(* Logix 5000 AddOnInstructionDefinition export SPEL_Above; software revision 30.01; part 3 of 9 *)

ADD_ON_INSTRUCTION SPEL_FineSet   (* revision 1.0, vendor SEIKO EPSON CORP. *)
// Sets the positioning end judgement range for all joints.
VAR_INPUT
   Start : BOOL; {required}
END_VAR
VAR_OUTPUT
   InCycle : BOOL; {access Read Only, visible}
   Done : BOOL; {access Read Only, visible}
   Error : BOOL; {access Read Only, visible}
END_VAR
VAR_INPUT
   Axis1 : DINT; {required}
   Axis2 : DINT; {required}
   Axis3 : DINT; {required}
   Axis4 : DINT; {required}
   Axis5 : DINT; {required}
   Axis6 : DINT; {required}
END_VAR
VAR_IN_OUT
   ExtInputs : AB:ETHERNET_MODULE_INT_128Bytes:I:0; {required}
   ExtOutputs : AB:ETHERNET_MODULE_INT_128Bytes:O:0; {required}
END_VAR
VAR_OUTPUT
   ErrCode1 : INT; {access Read Only, visible}
   ErrCode2 : INT; {access Read Only, visible}
END_VAR
VAR
   ExecFineSet : SPEL_ExecCmd := (MaxTime := 3000); {access None}
   OneShotStart : BOOL; {access None}
   StartCoil : BOOL; {access None}
   ExecTimeout : DINT; {access None}
END_VAR

ROUTINE Logic   (* ladder *)
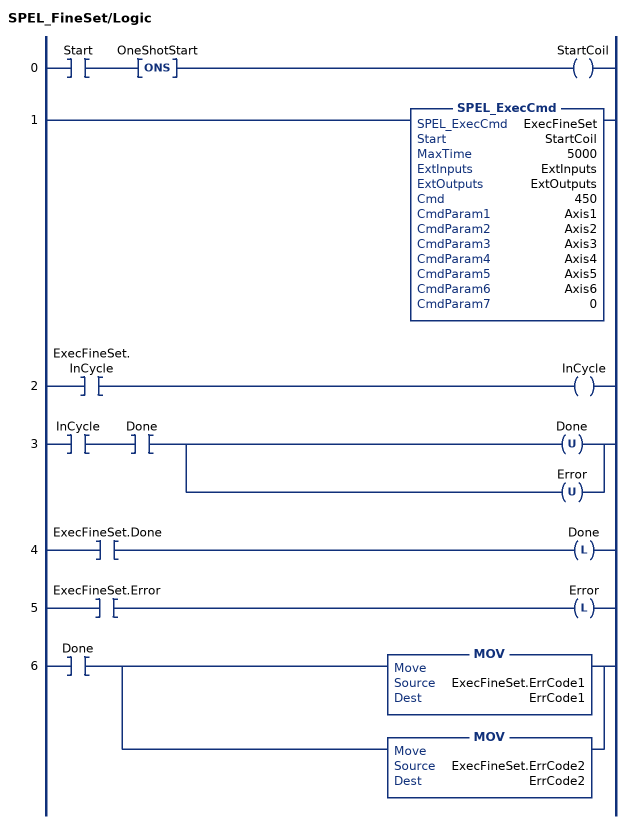
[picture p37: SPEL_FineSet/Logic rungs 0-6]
   0: XIC(Start)ONS(OneShotStart)OTE(StartCoil);
   1: SPEL_ExecCmd(ExecFineSet,StartCoil,5000,ExtInputs,ExtOutputs,450,Axis1,Axis2,Axis3,Axis4,Axis5,Axis6,0);
   2: XIC(ExecFineSet.InCycle)OTE(InCycle);
   3: XIC(InCycle)XIC(Done)[OTU(Done) ,OTU(Error) ];
   4: XIC(ExecFineSet.Done)OTL(Done);
   5: XIC(ExecFineSet.Error)OTL(Error);
   6: XIC(Done)[MOV(ExecFineSet.ErrCode1,ErrCode1) ,MOV(ExecFineSet.ErrCode2,ErrCode2) ];
END_ROUTINE
END_ADD_ON_INSTRUCTION

ADD_ON_INSTRUCTION SPEL_Flip   (* revision 1.0, vendor SEIKO EPSON CORP. *)
// Sets the wrist orientation of the specified point to Flip.
VAR_INPUT
   Start : BOOL; {required}
END_VAR
VAR_OUTPUT
   InCycle : BOOL; {access Read Only, visible}
   Done : BOOL; {access Read Only, visible}
   Error : BOOL; {access Read Only, visible}
END_VAR
VAR_INPUT
   Point : INT; {required}
END_VAR
VAR_IN_OUT
   ExtInputs : AB:ETHERNET_MODULE_INT_128Bytes:I:0; {required}
   ExtOutputs : AB:ETHERNET_MODULE_INT_128Bytes:O:0; {required}
END_VAR
VAR_OUTPUT
   ErrCode1 : INT; {access Read Only, visible}
   ErrCode2 : INT; {access Read Only, visible}
END_VAR
VAR
   ExecFlip : SPEL_ExecCmd := (MaxTime := 3000); {access None}
   OneShotStart : BOOL; {access None}
   StartCoil : BOOL; {access None}
   ExecTimeout : DINT; {access None}
END_VAR

ROUTINE Logic   (* ladder *)
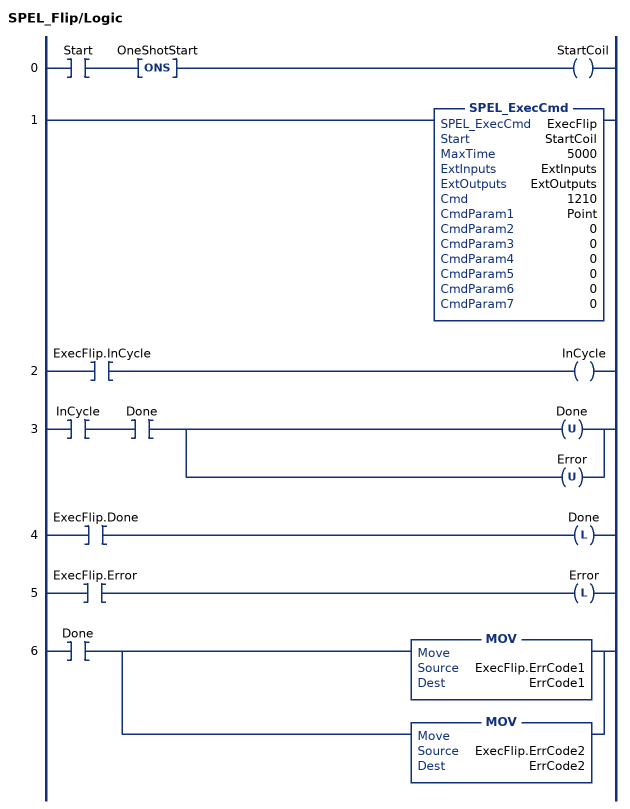
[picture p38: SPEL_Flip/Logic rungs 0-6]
   0: XIC(Start)ONS(OneShotStart)OTE(StartCoil);
   1: SPEL_ExecCmd(ExecFlip,StartCoil,5000,ExtInputs,ExtOutputs,1210,Point,0,0,0,0,0,0);
   2: XIC(ExecFlip.InCycle)OTE(InCycle);
   3: XIC(InCycle)XIC(Done)[OTU(Done) ,OTU(Error) ];
   4: XIC(ExecFlip.Done)OTL(Done);
   5: XIC(ExecFlip.Error)OTL(Error);
   6: XIC(Done)[MOV(ExecFlip.ErrCode1,ErrCode1) ,MOV(ExecFlip.ErrCode2,ErrCode2) ];
END_ROUTINE
END_ADD_ON_INSTRUCTION

ADD_ON_INSTRUCTION SPEL_Go   (* revision 1.0, vendor SEIKO EPSON CORP. *)
// Moves from the current position to the specified position in PTP motion.
VAR_INPUT
   Start : BOOL; {required}
   MaxTime : DINT := 30000; {access None, visible}
END_VAR
VAR_OUTPUT
   InCycle : BOOL; {access Read Only, visible}
   Done : BOOL; {access Read Only, visible}
   Error : BOOL; {access Read Only, visible}
END_VAR
VAR_INPUT
   TargetType : INT; {access None, visible}
   Point : INT; {required}
   PalletNum : INT; {access None, visible}
   PalletPosOrCol : INT; {access None, visible}
   PalletRow : INT; {access None, visible}
END_VAR
VAR_IN_OUT
   ExtInputs : AB:ETHERNET_MODULE_INT_128Bytes:I:0; {required}
   ExtOutputs : AB:ETHERNET_MODULE_INT_128Bytes:O:0; {required}
END_VAR
VAR_OUTPUT
   ErrCode1 : INT; {access Read Only, visible}
   ErrCode2 : INT; {access Read Only, visible}
END_VAR
VAR
   ExecGo : SPEL_ExecCmd := (MaxTime := 3000); {access None}
        .INCYCLE   // ExecInCycle
        .DONE   // ExecDone
        .ERROR   // ExecError
   OneShotStart : BOOL; {access None}
   StartInit : BOOL; {access None}
   JumpTargetType : INT; {access None}
   GoTargetType : INT; {access None}
   PointOrPalletNum : INT; {access None}
   ExecTimeout : DINT; {access None}
   OneShotCP : BOOL; {access None}
   LocalCP : DINT; {access None}
   CmdParam1 : DINT; {access None}
   TargetTypeError : BOOL; {access None}
   StartExec : BOOL; {access None}
   ExecuteCmd : BOOL; {access None}
   OneShotTargetType : BOOL; {access None}
END_VAR

ROUTINE Logic   (* ladder *)
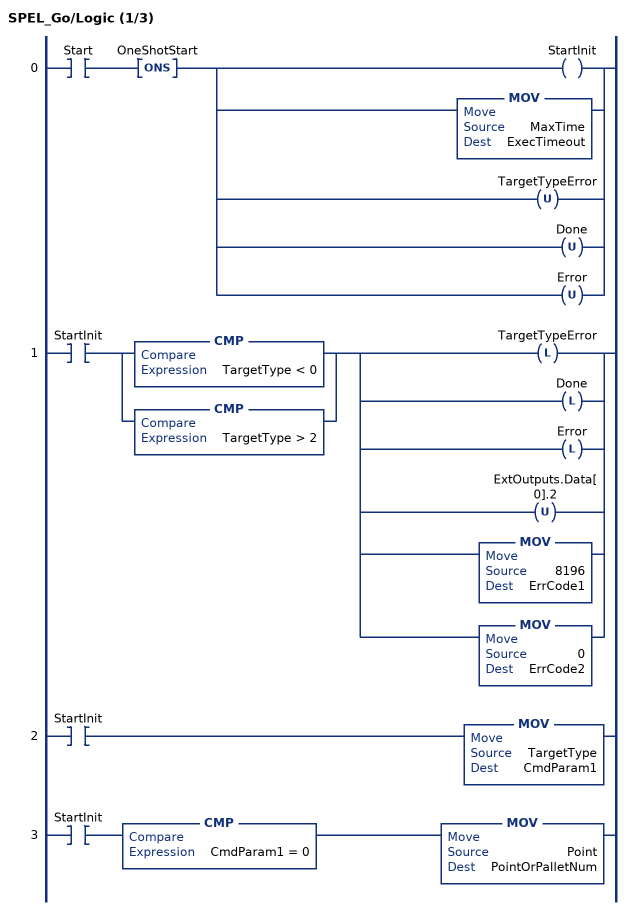
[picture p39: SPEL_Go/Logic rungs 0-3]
   0: XIC(Start)ONS(OneShotStart)[OTE(StartInit) ,MOV(MaxTime,ExecTimeout) ,OTU(TargetTypeError) ,OTU(Done) ,OTU(Error) ];
   1: XIC(StartInit)[CMP(TargetType < 0) ,CMP(TargetType > 2) ][OTL(TargetTypeError) ,OTL(Done) ,OTL(Error) ,OTU(ExtOutputs.Data[0].2) ,MOV(8196,ErrCode1) ,MOV(0,ErrCode2) ];
   2: XIC(StartInit)MOV(TargetType,CmdParam1);
   3: XIC(StartInit)CMP(CmdParam1 = 0)MOV(Point,PointOrPalletNum);
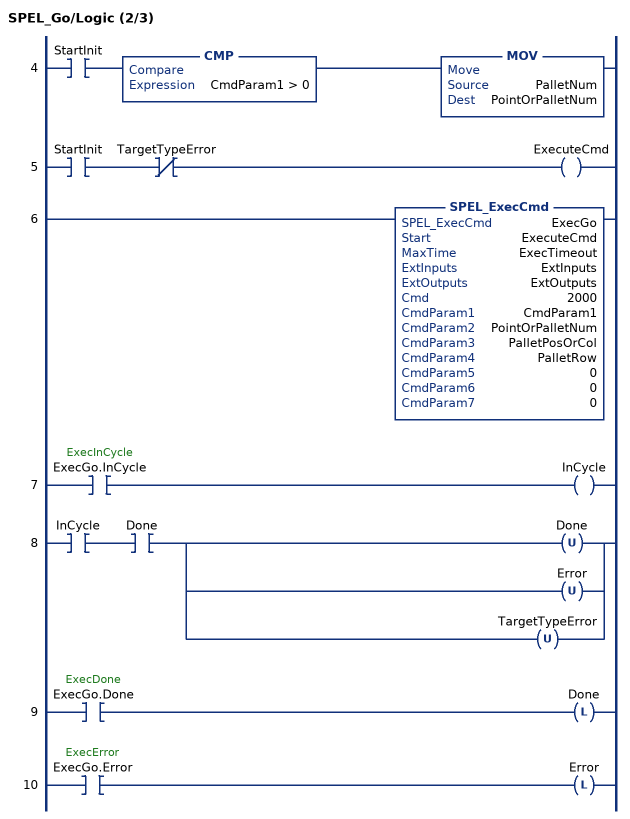
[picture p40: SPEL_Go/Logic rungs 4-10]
   4: XIC(StartInit)CMP(CmdParam1 > 0)MOV(PalletNum,PointOrPalletNum);
   5: XIC(StartInit)XIO(TargetTypeError)OTE(ExecuteCmd);
   6: SPEL_ExecCmd(ExecGo,ExecuteCmd,ExecTimeout,ExtInputs,ExtOutputs,2000,CmdParam1,PointOrPalletNum,PalletPosOrCol,PalletRow,0,0,0);
   7: XIC(ExecGo.InCycle)OTE(InCycle);
   8: XIC(InCycle)XIC(Done)[OTU(Done) ,OTU(Error) ,OTU(TargetTypeError) ];
   9: XIC(ExecGo.Done)OTL(Done);
   10: XIC(ExecGo.Error)OTL(Error);
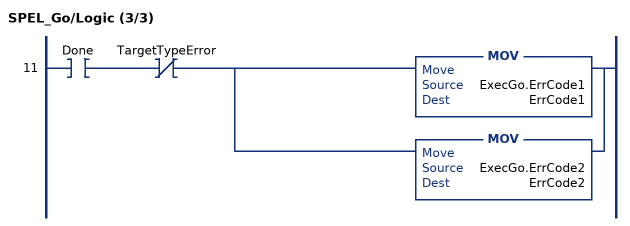
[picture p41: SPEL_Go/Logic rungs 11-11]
   11: XIC(Done)XIO(TargetTypeError)[MOV(ExecGo.ErrCode1,ErrCode1) ,MOV(ExecGo.ErrCode2,ErrCode2) ];
END_ROUTINE
END_ADD_ON_INSTRUCTION

ADD_ON_INSTRUCTION SPEL_In   (* revision 1.0, vendor SEIKO EPSON CORP. *)
// Reads a byte of input.
VAR_INPUT
   Start : BOOL; {access Read Only, required}
END_VAR
VAR_OUTPUT
   InCycle : BOOL; {access Read Only, visible}
   Done : BOOL; {access Read Only, visible}
   Error : BOOL; {access Read Only, visible}
END_VAR
VAR_INPUT
   PortNum : INT; {required}
END_VAR
VAR_OUTPUT
   Value : INT; {access Read Only, visible}
END_VAR
VAR_IN_OUT
   ExtInputs : AB:ETHERNET_MODULE_INT_128Bytes:I:0; {required}
   ExtOutputs : AB:ETHERNET_MODULE_INT_128Bytes:O:0; {required}
END_VAR
VAR_OUTPUT
   ErrCode1 : INT; {access Read Only, visible}
   ErrCode2 : INT; {access Read Only, visible}
END_VAR
VAR
   ExeIn : SPEL_ExecCmd := (MaxTime := 3000); {access None}
        .INCYCLE   // ExecInCycle
        .DONE   // ExecDone
        .ERROR   // ExecError
   OneShotStart : BOOL; {access None}
   StartCoil : BOOL; {access None}
   ExecTimeout : DINT; {access None}
END_VAR

ROUTINE Logic   (* ladder *)
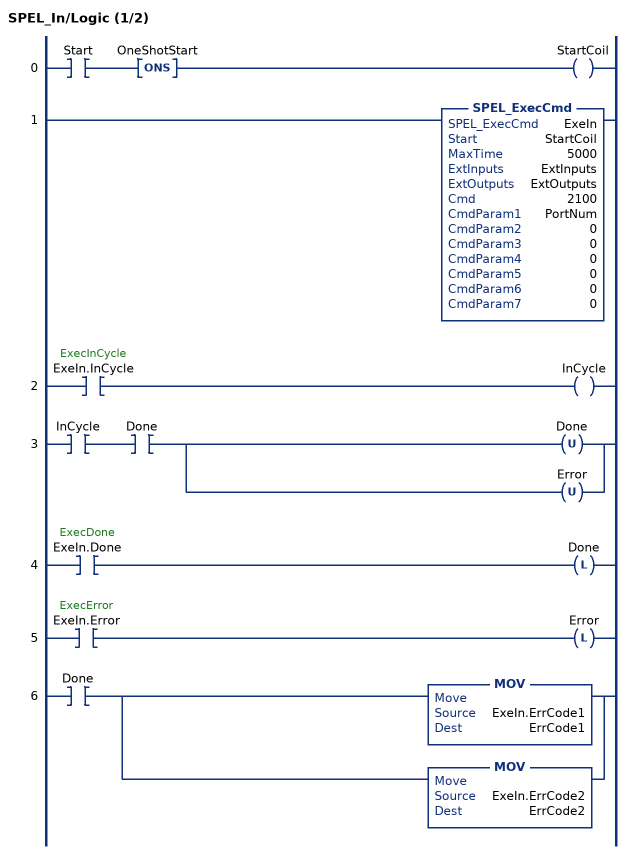
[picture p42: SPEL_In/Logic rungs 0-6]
   0: XIC(Start)ONS(OneShotStart)OTE(StartCoil);
   1: SPEL_ExecCmd(ExeIn,StartCoil,5000,ExtInputs,ExtOutputs,2100,PortNum,0,0,0,0,0,0);
   2: XIC(ExeIn.InCycle)OTE(InCycle);
   3: XIC(InCycle)XIC(Done)[OTU(Done) ,OTU(Error) ];
   4: XIC(ExeIn.Done)OTL(Done);
   5: XIC(ExeIn.Error)OTL(Error);
   6: XIC(Done)[MOV(ExeIn.ErrCode1,ErrCode1) ,MOV(ExeIn.ErrCode2,ErrCode2) ];
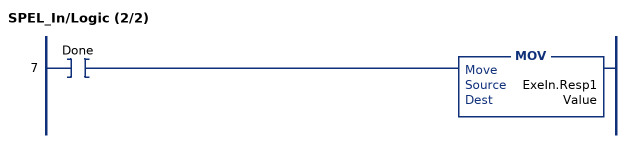
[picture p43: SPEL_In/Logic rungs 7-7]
   7: XIC(Done)MOV(ExeIn.Resp1,Value);
END_ROUTINE
END_ADD_ON_INSTRUCTION

ADD_ON_INSTRUCTION SPEL_InW   (* revision 1.0, vendor SEIKO EPSON CORP. *)
// Returns the status if an input word.
VAR_INPUT
   Start : BOOL; {access Read Only, required}
END_VAR
VAR_OUTPUT
   InCycle : BOOL; {access Read Only, visible}
   Done : BOOL; {access Read Only, visible}
   Error : BOOL; {access Read Only, visible}
END_VAR
VAR_INPUT
   PortNum : INT; {required}
END_VAR
VAR_OUTPUT
   Value : DINT; {access Read Only, visible}
END_VAR
VAR_IN_OUT
   ExtInputs : AB:ETHERNET_MODULE_INT_128Bytes:I:0; {required}
   ExtOutputs : AB:ETHERNET_MODULE_INT_128Bytes:O:0; {required}
END_VAR
VAR_OUTPUT
   ErrCode1 : INT; {access Read Only, visible}
   ErrCode2 : INT; {access Read Only, visible}
END_VAR
VAR
   ExeInW : SPEL_ExecCmd := (MaxTime := 3000); {access None}
        .INCYCLE   // ExecInCycle
        .DONE   // ExecDone
        .ERROR   // ExecError
   OneShotStart : BOOL; {access None}
   StartCoil : BOOL; {access None}
   ExecTimeout : DINT; {access None}
END_VAR

ROUTINE Logic   (* ladder *)
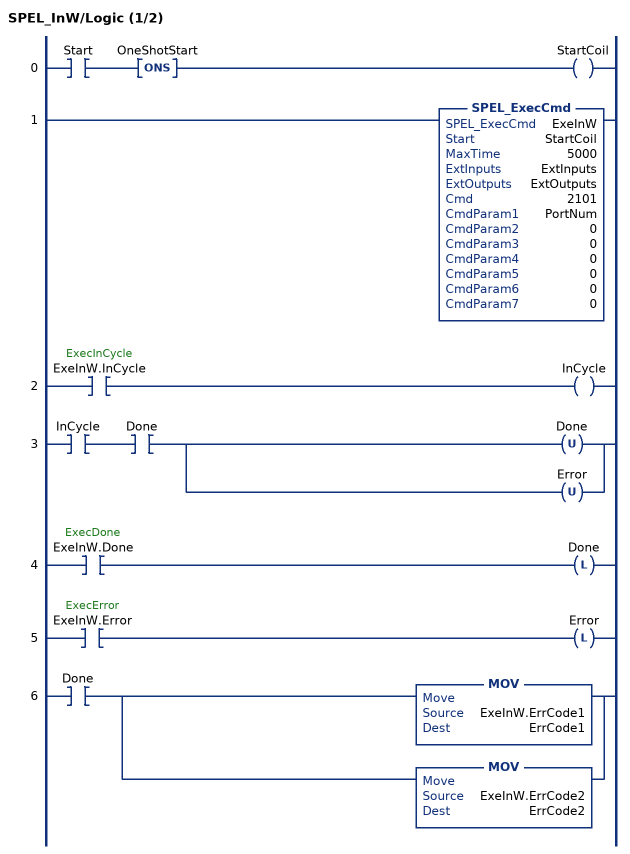
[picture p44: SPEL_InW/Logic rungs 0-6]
   0: XIC(Start)ONS(OneShotStart)OTE(StartCoil);
   1: SPEL_ExecCmd(ExeInW,StartCoil,5000,ExtInputs,ExtOutputs,2101,PortNum,0,0,0,0,0,0);
   2: XIC(ExeInW.InCycle)OTE(InCycle);
   3: XIC(InCycle)XIC(Done)[OTU(Done) ,OTU(Error) ];
   4: XIC(ExeInW.Done)OTL(Done);
   5: XIC(ExeInW.Error)OTL(Error);
   6: XIC(Done)[MOV(ExeInW.ErrCode1,ErrCode1) ,MOV(ExeInW.ErrCode2,ErrCode2) ];
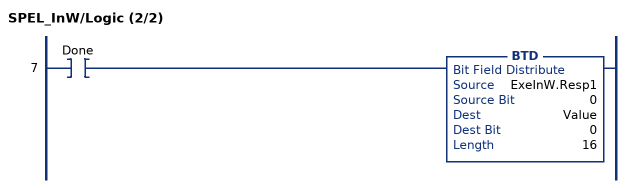
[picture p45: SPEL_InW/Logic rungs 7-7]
   7: XIC(Done)BTD(ExeInW.Resp1,0,Value,0,16);
END_ROUTINE
END_ADD_ON_INSTRUCTION

ADD_ON_INSTRUCTION SPEL_InertiaGet   (* revision 1.0, vendor SEIKO EPSON CORP. *)
// Gets the load inertia.
VAR_INPUT
   Start : BOOL; {required}
END_VAR
VAR_OUTPUT
   InCycle : BOOL; {access Read Only, visible}
   Done : BOOL; {access Read Only, visible}
   Error : BOOL; {access Read Only, visible}
   Inertia : REAL; {visible}
   Eccentricity : REAL; {visible}
END_VAR
VAR_IN_OUT
   ExtInputs : AB:ETHERNET_MODULE_INT_128Bytes:I:0; {required}
   ExtOutputs : AB:ETHERNET_MODULE_INT_128Bytes:O:0; {required}
END_VAR
VAR_OUTPUT
   ErrCode1 : DINT; {access Read Only, visible}
   ErrCode2 : DINT; {access Read Only, visible}
END_VAR
VAR
   ExecInertiaGet : SPEL_ExecCmd := (MaxTime := 3000); {access None}
   Inertiax1000 : DINT; {access None}
   Inertia_INTS : INT[2]; {access None}
   Eccentricityx1000 : DINT; {access None}
   Eccentricity_INTS : INT[2]; {access None}
   OneShotStart : BOOL; {access None}
   StartCoil : BOOL; {access None}
   ExecTimeout : DINT; {access None}
END_VAR

ROUTINE Logic   (* ladder *)
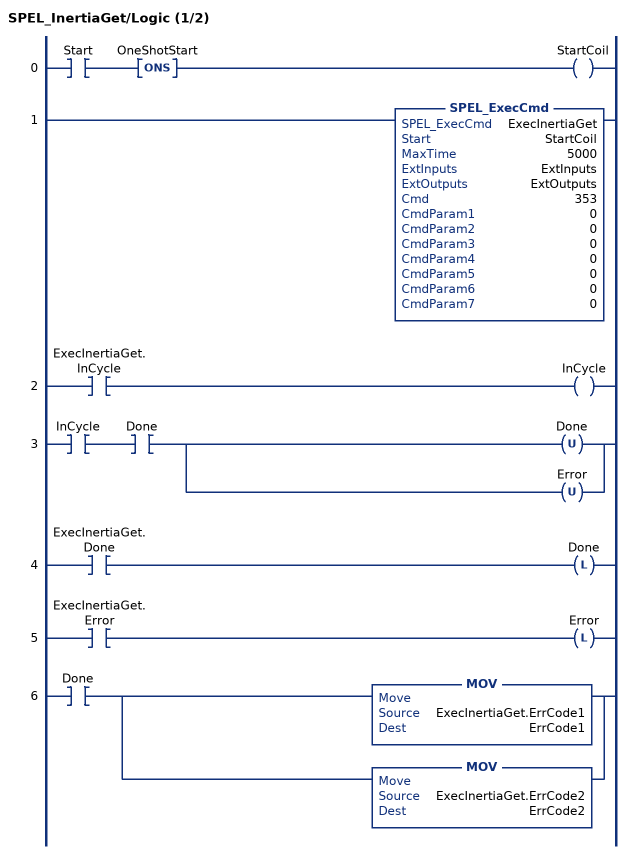
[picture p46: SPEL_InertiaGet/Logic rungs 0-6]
   0: XIC(Start)ONS(OneShotStart)OTE(StartCoil);
   1: SPEL_ExecCmd(ExecInertiaGet,StartCoil,5000,ExtInputs,ExtOutputs,353,0,0,0,0,0,0,0);
   2: XIC(ExecInertiaGet.InCycle)OTE(InCycle);
   3: XIC(InCycle)XIC(Done)[OTU(Done) ,OTU(Error) ];
   4: XIC(ExecInertiaGet.Done)OTL(Done);
   5: XIC(ExecInertiaGet.Error)OTL(Error);
   6: XIC(Done)[MOV(ExecInertiaGet.ErrCode1,ErrCode1) ,MOV(ExecInertiaGet.ErrCode2,ErrCode2) ];
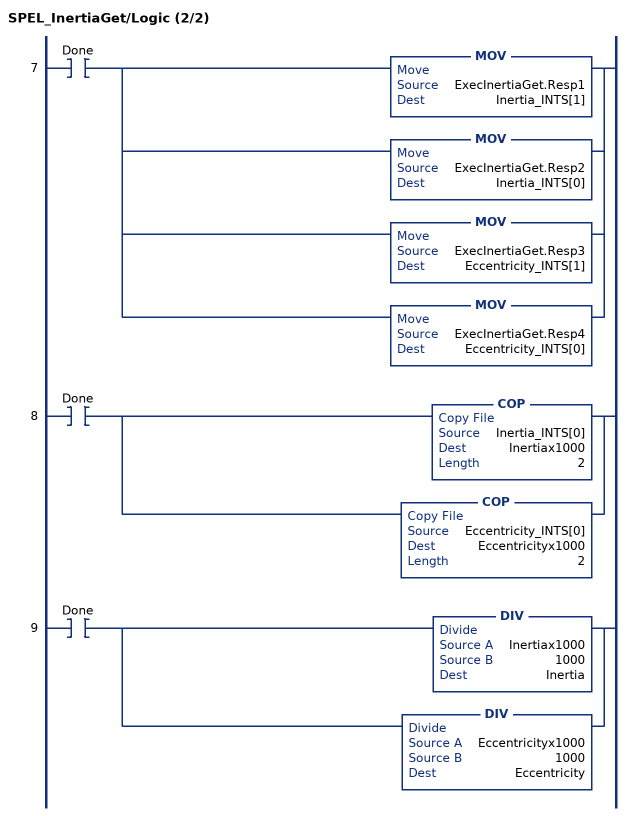
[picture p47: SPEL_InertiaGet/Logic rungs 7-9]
   7: XIC(Done)[MOV(ExecInertiaGet.Resp1,Inertia_INTS[1]) ,MOV(ExecInertiaGet.Resp2,Inertia_INTS[0]) ,MOV(ExecInertiaGet.Resp3,Eccentricity_INTS[1]) ,MOV(ExecInertiaGet.Resp4,Eccentricity_INTS[0]) ];
   8: XIC(Done)[COP(Inertia_INTS[0],Inertiax1000,2) ,COP(Eccentricity_INTS[0],Eccentricityx1000,2) ];
   9: XIC(Done)[DIV(Inertiax1000,1000,Inertia) ,DIV(Eccentricityx1000,1000,Eccentricity) ];
END_ROUTINE
END_ADD_ON_INSTRUCTION

ADD_ON_INSTRUCTION SPEL_InertiaSet   (* revision 1.0, vendor SEIKO EPSON CORP. *)
// Sets the load inertia.
VAR_INPUT
   Start : BOOL; {required}
END_VAR
VAR_OUTPUT
   InCycle : BOOL; {access Read Only, visible}
   Done : BOOL; {access Read Only, visible}
   Error : BOOL; {access Read Only, visible}
END_VAR
VAR_INPUT
   Inertia : REAL; {required}
   Eccentricity : REAL; {required}
END_VAR
VAR_IN_OUT
   ExtInputs : AB:ETHERNET_MODULE_INT_128Bytes:I:0; {required}
   ExtOutputs : AB:ETHERNET_MODULE_INT_128Bytes:O:0; {required}
END_VAR
VAR_OUTPUT
   ErrCode1 : INT; {access Read Only, visible}
   ErrCode2 : INT; {access Read Only, visible}
END_VAR
VAR
   StartInit : BOOL; {access None}
   OneShotStart : BOOL; {access None}
   ExecInertiaSet : SPEL_ExecCmd := (MaxTime := 3000); {access None}
   Inertiax1000 : DINT; {access None}
   Inertia_INTS : INT[2]; {access None}
   Eccentricityx1000 : DINT; {access None}
   Eccentricity_INTS : INT[2]; {access None}
   ExecTimeout : DINT; {access None}
END_VAR

ROUTINE Logic   (* ladder *)
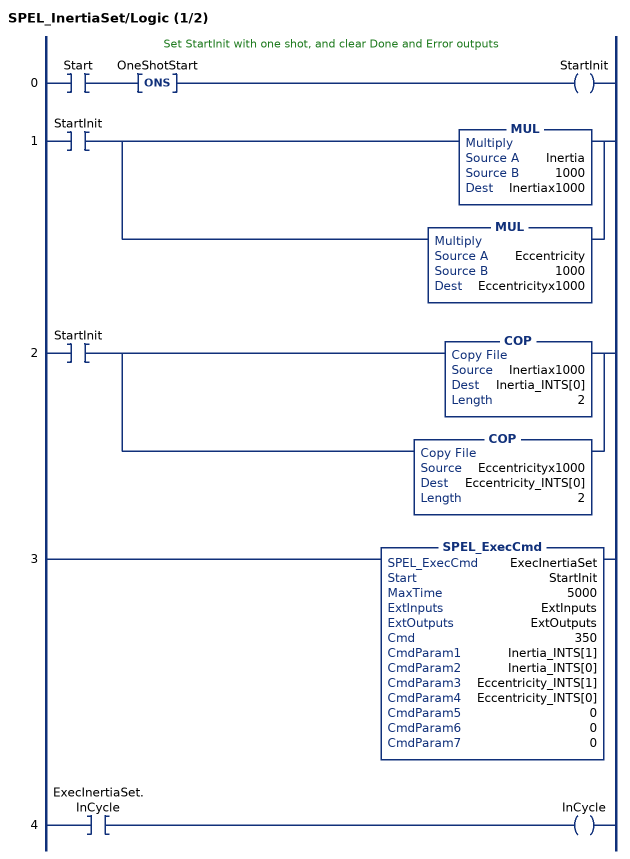
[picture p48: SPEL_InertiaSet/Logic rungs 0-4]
   // Set StartInit with one shot, and clear Done and Error outputs
   0: XIC(Start)ONS(OneShotStart)OTE(StartInit);
   1: XIC(StartInit)[MUL(Inertia,1000,Inertiax1000) ,MUL(Eccentricity,1000,Eccentricityx1000) ];
   2: XIC(StartInit)[COP(Inertiax1000,Inertia_INTS[0],2) ,COP(Eccentricityx1000,Eccentricity_INTS[0],2) ];
   3: SPEL_ExecCmd(ExecInertiaSet,StartInit,5000,ExtInputs,ExtOutputs,350,Inertia_INTS[1],Inertia_INTS[0],Eccentricity_INTS[1],Eccentricity_INTS[0],0,0,0);
   4: XIC(ExecInertiaSet.InCycle)OTE(InCycle);
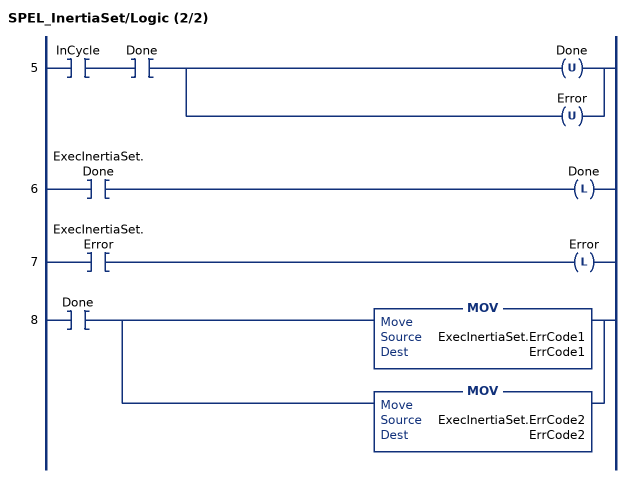
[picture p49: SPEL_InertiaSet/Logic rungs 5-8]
   5: XIC(InCycle)XIC(Done)[OTU(Done) ,OTU(Error) ];
   6: XIC(ExecInertiaSet.Done)OTL(Done);
   7: XIC(ExecInertiaSet.Error)OTL(Error);
   8: XIC(Done)[MOV(ExecInertiaSet.ErrCode1,ErrCode1) ,MOV(ExecInertiaSet.ErrCode2,ErrCode2) ];
END_ROUTINE
END_ADD_ON_INSTRUCTION

ADD_ON_INSTRUCTION SPEL_ResetError   (* revision 1.0 *)
// Resets AOI library error state. This AOI must be executed to clear an error.
VAR_OUTPUT
   InCycle : BOOL; {access Read Only, visible}
   Done : BOOL; {visible}
   Error : BOOL; {access Read Only, visible}
END_VAR
VAR_INPUT
   Start : BOOL; {required}
END_VAR
VAR_IN_OUT
   ExtInputs : AB:ETHERNET_MODULE_INT_128Bytes:I:0; {required}
   ExtOutputs : AB:ETHERNET_MODULE_INT_128Bytes:O:0; {required}
END_VAR
VAR_OUTPUT
   ErrCode1 : INT; {access Read Only, visible}
   ErrCode2 : INT; {access Read Only, visible}
END_VAR
VAR
   TmrReset : TIMER := (PRE := 50); {access None}
   OneShotStart : BOOL; {access None}
   OneShotStart1 : BOOL; {access None}
   StartInit : BOOL; {access None}
   TmrWaitRdy : TIMER := (PRE := 100); {access None}
END_VAR

ROUTINE Logic   (* ladder *)
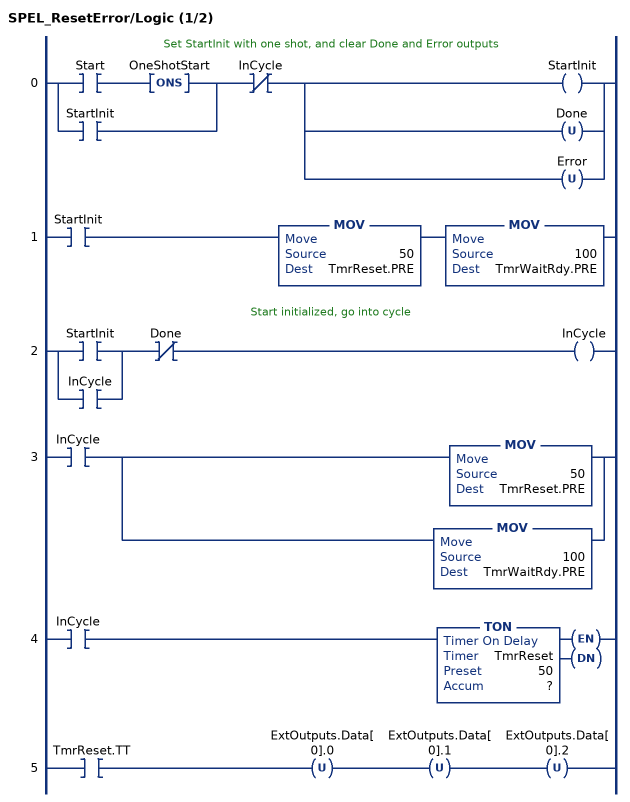
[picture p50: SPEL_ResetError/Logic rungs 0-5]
   // Set StartInit with one shot, and clear Done and Error outputs
   0: [XIC(Start) ONS(OneShotStart) ,XIC(StartInit) ]XIO(InCycle)[OTE(StartInit) ,[OTU(Done) ,OTU(Error) ] ];
   1: XIC(StartInit)MOV(50,TmrReset.PRE)MOV(100,TmrWaitRdy.PRE);
   // Start initialized, go into cycle
   2: [XIC(StartInit) ,XIC(InCycle) ]XIO(Done)OTE(InCycle);
   3: XIC(InCycle)[MOV(50,TmrReset.PRE) ,MOV(100,TmrWaitRdy.PRE) ];
   4: XIC(InCycle)TON(TmrReset,?,?);
   5: XIC(TmrReset.TT)OTU(ExtOutputs.Data[0].0)OTU(ExtOutputs.Data[0].1)OTU(ExtOutputs.Data[0].2);
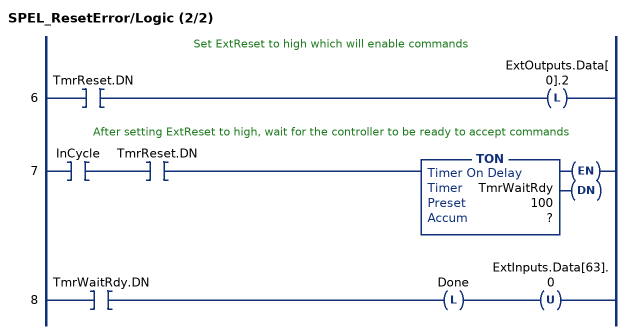
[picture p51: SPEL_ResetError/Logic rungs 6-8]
   // Set ExtReset to high which will enable commands
   6: XIC(TmrReset.DN)OTL(ExtOutputs.Data[0].2);
   // After setting ExtReset to high, wait for the controller to be ready to accept commands
   7: XIC(InCycle)XIC(TmrReset.DN)TON(TmrWaitRdy,?,?);
   8: XIC(TmrWaitRdy.DN)OTL(Done)OTU(ExtInputs.Data[63].0);
END_ROUTINE
END_ADD_ON_INSTRUCTION

ADD_ON_INSTRUCTION SPEL_Init   (* revision 1.0 *)
// Initialize the SPEL AOI library.
VAR_INPUT
   Start : BOOL; {required}
END_VAR
VAR_OUTPUT
   InCycle : BOOL; {access Read Only, visible}
   Done : BOOL; {access Read Only, visible}
   Error : BOOL; {access Read Only, visible}
END_VAR
VAR_IN_OUT
   ExtInputs : AB:ETHERNET_MODULE_INT_128Bytes:I:0; {required}
   ExtOutputs : AB:ETHERNET_MODULE_INT_128Bytes:O:0; {required}
END_VAR
VAR_OUTPUT
   ErrCode1 : INT; {access Read Only, visible}
   ErrCode2 : INT; {access Read Only, visible}
END_VAR
VAR
   ResetError : SPEL_ResetError; {access None}
        .INCYCLE   // ResetErrorInCycle
   ExecGetCCD : SPEL_ExecCmd := (MaxTime := 3000); {access None}
   RemoteIO_OK : BOOL; {access None}
   ExecGetPLC_ID : SPEL_ExecCmd := (MaxTime := 3000); {access None}
   AB_OK : BOOL; {access None}
   RemoteIO_Err : BOOL; {access None}
   AB_Err : BOOL; {access None}
   StartGetCCD : BOOL; {access None}
   StartGetCD_ONS : BOOL; {access None}
   Disable : BOOL; {access None}
   Disable2 : BOOL; {access None}
   TestStartCD : BOOL; {access None}
   TmrStartGetCD : TIMER := (PRE := 50); {access None}
   OneShotStartGetCCD : BOOL; {access None}
   StartGetPLC : BOOL; {access None}
   OneShotStartGetPLC : BOOL; {access None}
   ExecTimeout : DINT; {access None}
END_VAR

ROUTINE Logic   (* ladder *)
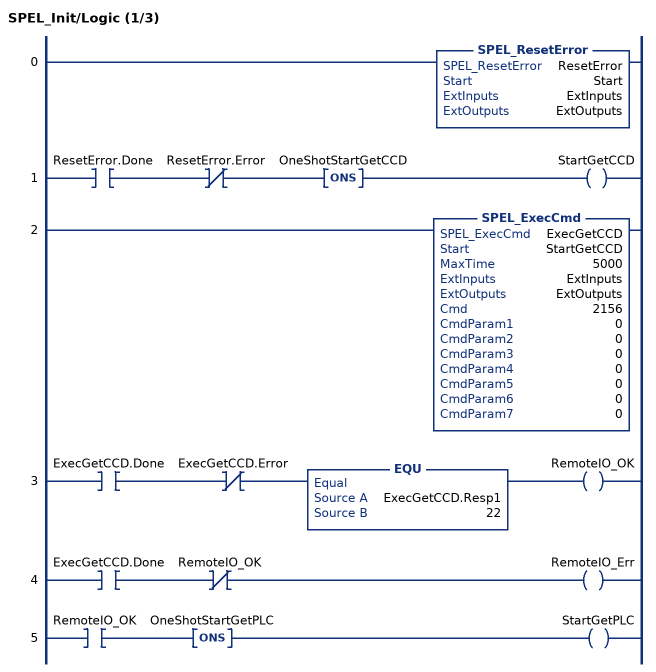
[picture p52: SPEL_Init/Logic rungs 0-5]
   0: SPEL_ResetError(ResetError,Start,ExtInputs,ExtOutputs);
   1: XIC(ResetError.Done)XIO(ResetError.Error)ONS(OneShotStartGetCCD)OTE(StartGetCCD);
   2: SPEL_ExecCmd(ExecGetCCD,StartGetCCD,5000,ExtInputs,ExtOutputs,2156,0,0,0,0,0,0,0);
   3: XIC(ExecGetCCD.Done)XIO(ExecGetCCD.Error)EQU(ExecGetCCD.Resp1,22)OTE(RemoteIO_OK);
   4: XIC(ExecGetCCD.Done)XIO(RemoteIO_OK)OTE(RemoteIO_Err);
   5: XIC(RemoteIO_OK)ONS(OneShotStartGetPLC)OTE(StartGetPLC);
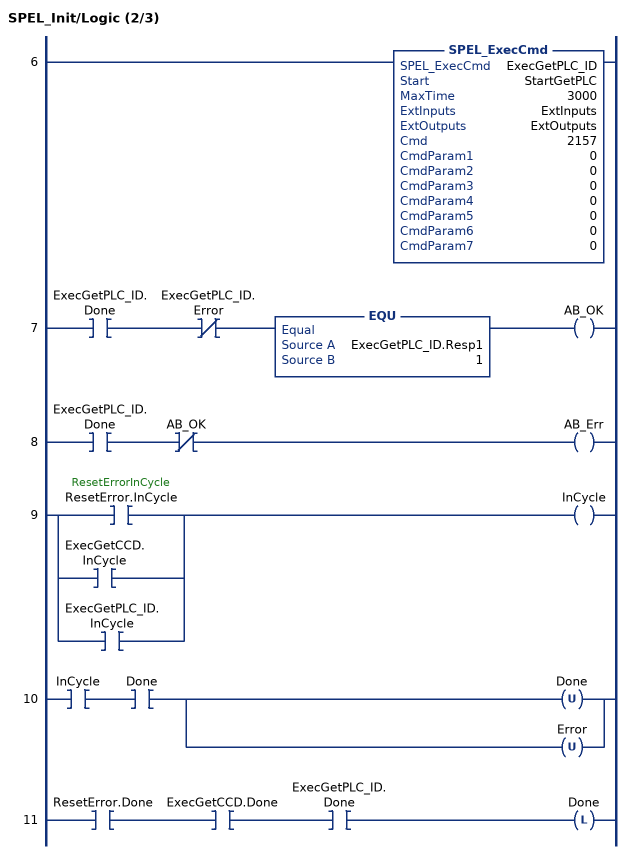
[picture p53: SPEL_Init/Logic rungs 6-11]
   6: SPEL_ExecCmd(ExecGetPLC_ID,StartGetPLC,3000,ExtInputs,ExtOutputs,2157,0,0,0,0,0,0,0);
   7: XIC(ExecGetPLC_ID.Done)XIO(ExecGetPLC_ID.Error)EQU(ExecGetPLC_ID.Resp1,1)OTE(AB_OK);
   8: XIC(ExecGetPLC_ID.Done)XIO(AB_OK)OTE(AB_Err);
   9: [XIC(ResetError.InCycle) ,XIC(ExecGetCCD.InCycle) ,XIC(ExecGetPLC_ID.InCycle) ]OTE(InCycle);
   10: XIC(InCycle)XIC(Done)[OTU(Done) ,OTU(Error) ];
   11: XIC(ResetError.Done)XIC(ExecGetCCD.Done)XIC(ExecGetPLC_ID.Done)OTL(Done);
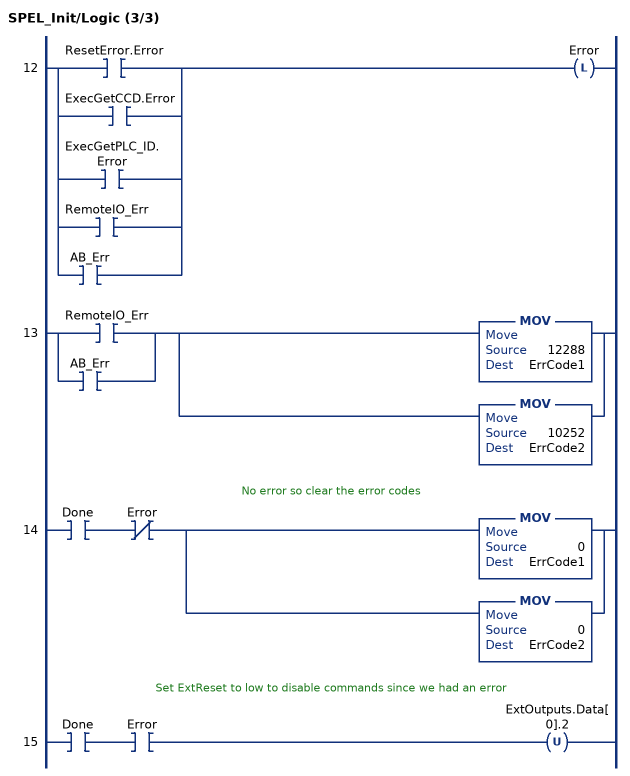
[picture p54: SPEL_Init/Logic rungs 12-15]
   12: [XIC(ResetError.Error) ,XIC(ExecGetCCD.Error) ,XIC(ExecGetPLC_ID.Error) ,XIC(RemoteIO_Err) ,XIC(AB_Err) ]OTL(Error);
   13: [XIC(RemoteIO_Err) ,XIC(AB_Err) ][MOV(12288,ErrCode1) ,MOV(10252,ErrCode2) ];
   // No error so clear the error codes
   14: XIC(Done)XIO(Error)[MOV(0,ErrCode1) ,MOV(0,ErrCode2) ];
   // Set ExtReset to low to disable commands since we had an error
   15: XIC(Done)XIC(Error)OTU(ExtOutputs.Data[0].2);
END_ROUTINE
END_ADD_ON_INSTRUCTION
